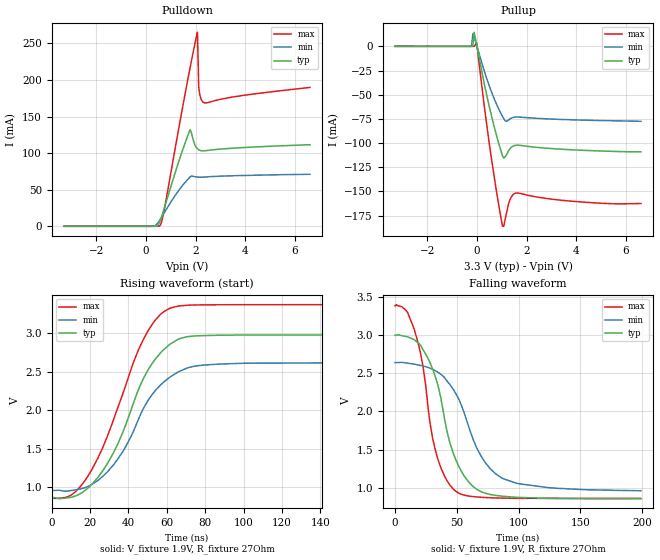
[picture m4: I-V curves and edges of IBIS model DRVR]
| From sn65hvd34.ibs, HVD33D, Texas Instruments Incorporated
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|   Driver Output / Receiver Input Model
[Model]   DRVR
Model_type   3-state
|Signal   Z,Y
Polarity   Non-Inverting
Enable   Active-Low
Vmeas = 2.09
Cref  = 50pF
Rref  = 27
| variable   typ   min   max
C_comp   535.9fF   508.7fF   548.1fF
|C_comp (Low state)   522.4fF   477.9fF   539.1fF
|C_comp (OFF state)   37.8pF   38.1pF   38.6pF
|   typ   min   max
[Voltage Range]   3.3   3   3.6
[Temperature Range]   27   85   -40
[Pullup Reference]   3.3   3   3.6
[Pulldown Reference]   -0   -0   -0
[Power Clamp Reference]   3.3   3   3.6
[GND Clamp Reference]   -0   -0   -0
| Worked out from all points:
|   slope of the pulldown table from 0 to 0.495 V, typ, clamps not added: 206 ohm
|   slope of the pullup table from 0 to 0.495 V, typ, clamps not added: 7.96 ohm
|   falling waveform, V_fixture 1.9V, R_fixture 27Ohm: 20-80 % time 21.4ns typ, 28.2ns min, 16ns max; typ from 2.99 V to 0.86 V
|   rising waveform, V_fixture 1.9V, R_fixture 27Ohm: 20-80 % time 22.6ns typ, 23.1ns min, 23ns max; typ from 0.86 V to 2.98 V
[Pulldown]
|   Voltage   I(typ)   I(min)   I(max)
-3.3V     -74.6pA    -28.97nA   -61.67pA
281.9mV   2.074uA    96.36uA    2.386nA
480.9mV   1.606mA    4.79mA     24.87uA
580.4mV   8.506mA    9.847mA    1.675mA
729.6mV   23.91mA    18.15mA    21.69mA
1.774V    132.1mA    67.49mA    216.4mA
1.973V    110.9mA    67.81mA    250.3mA
2.073V    105.9mA    67.31mA    265.2mA
2.123V    104.6mA    67.17mA    190.6mA
2.222V    103.4mA    67.09mA    173.5mA
2.322V    103.2mA    67.23mA    169.2mA
6.6V      111.6mA    71.13mA    189.9mA
[Pullup]
|   Voltage   I(typ)   I(min)   I(max)
-3.3V     18.67uA    17.08uA    20.37uA
-215.6mV  2.047uA    1.89uA     2.349uA
-165.8mV  2.036uA    13.06mA    2.343uA
-116.1mV  14.55mA    9.497mA    2.332uA
-16.58mV  2.324mA    1.537mA    3.717mA
530.7mV   -66mA      -43.33mA   -106.5mA
1.028V    -113.1mA   -72.45mA   -186.1mA
1.078V    -115.5mA   -74.75mA   -186mA
1.327V    -105.9mA   -75.02mA   -158.7mA
1.575V    -102.2mA   -73.06mA   -151.7mA
3.864V    -107mA     -75.99mA   -160.2mA
6.6V      -109mA     -77.51mA   -162.5mA
[Ramp]
R_load = 27
|   typ   min   max
dV/dt_r   1.26907/2.25489e-08   0.995714/2.29997e-08   1.50202/2.30048e-08
dV/dt_f   1.28009/2.13503e-08   1.00438/2.80867e-08   1.50991/1.59373e-08
[Falling Waveform]
V_fixture = 1.9V
V_fixture_min = 1.795V
V_fixture_max = 2.12V
R_fixture = 27Ohm
C_fixture = 0F
|   Time   V(typ)   V(min)   V(max)
0s        2.994V     2.637V     3.38V
9.4ns     2.977V     2.632V     3.309V
15.9ns    2.933V     2.616V     3.056V
22.4ns    2.814V     2.594V     2.61V
27.1ns    2.679V     2.572V     2.002V
36.1ns    2.25V      2.497V     1.31V
49ns      1.377V     2.239V     959.7mV
69.4ns    953.5mV    1.423V     879mV
87.1ns    892mV      1.124V     867.6mV
198.9ns   860.2mV    963.3mV    863.8mV
[Rising Waveform]
V_fixture = 1.9V
V_fixture_min = 1.795V
V_fixture_max = 2.12V
R_fixture = 27Ohm
C_fixture = 0F
|   Time   V(typ)   V(min)   V(max)
0s        860.1mV    958.6mV    863.7mV
12.3ns    885.2mV    965.7mV    939.8mV
24.2ns    1.132V     1.091V     1.384V
37ns      1.707V     1.461V     2.207V
46.9ns    2.362V     1.976V     2.871V
53.8ns    2.655V     2.247V     3.161V
60.5ns    2.831V     2.407V     3.307V
70.5ns    2.951V     2.545V     3.359V
86.9ns    2.971V     2.596V     3.366V
198.9ns   2.975V     2.618V     3.367V
